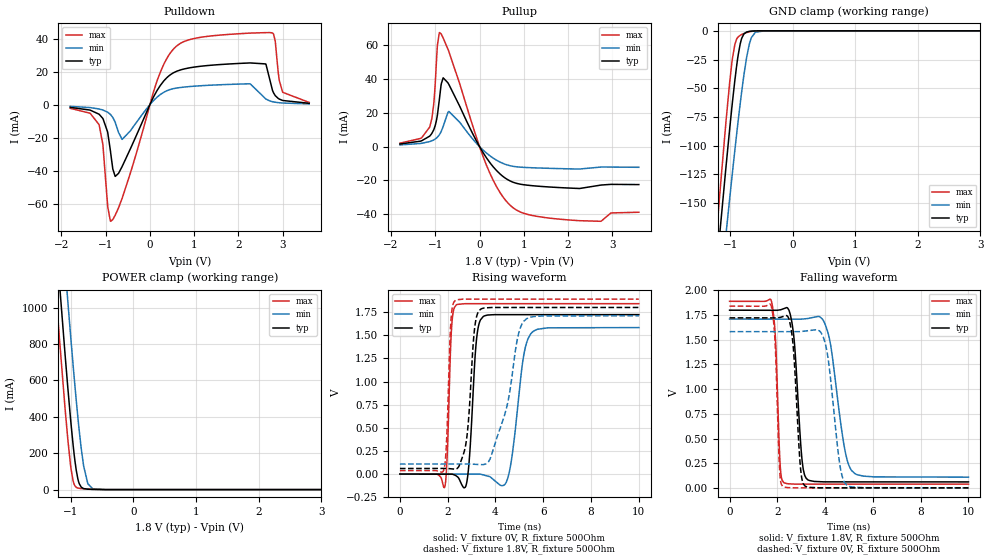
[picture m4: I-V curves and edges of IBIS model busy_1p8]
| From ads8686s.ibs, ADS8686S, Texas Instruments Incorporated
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|   busy_1p8 Model
[Model]   busy_1p8
Model_type   3-state
Polarity   Non-Inverting
Vmeas = 0.9
Vref = 0.9
Cref = 15pF
Rref = 50
|   typ   min   max
C_comp   1.54pF   1.54pF   1.57pF
[Voltage Range]   1.8   1.71   1.89
[Temperature Range]   27   125   -40
[Pullup Reference]   1.8   1.71   1.89
[Pulldown Reference]   0   0   0
[Power Clamp Reference]   1.8   1.71   1.89
[GND Clamp Reference]   0   0   0
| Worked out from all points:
|   slope of the pulldown table from 0 to 0.27 V, typ, clamps not added: 21 ohm
|   slope of the pullup table from 0 to 0.27 V, typ, clamps not added: 25.2 ohm
|   GND clamp passes 1 mA (typ) near -0.73 V on its own axis
|   POWER clamp passes 1 mA (typ) near -0.62 V on its own axis
|   falling waveform, V_fixture 1.8V, R_fixture 500Ohm: 20-80 % time 269ps typ, 526ps min, 163ps max; typ from 1.8 V to 0.06 V
|   rising waveform, V_fixture 0V, R_fixture 500Ohm: 20-80 % time 225ps typ, 418ps min, 136ps max; typ from 0 V to 1.72 V
|   rising waveform, V_fixture 1.8V, R_fixture 500Ohm: 20-80 % time 275ps typ, 761ps min, 144ps max; typ from 0.06 V to 1.8 V
|   falling waveform, V_fixture 0V, R_fixture 500Ohm: 20-80 % time 242ps typ, 420ps min, 155ps max; typ from 1.72 V to 0 V
[Pulldown]
|   Voltage   I(typ)   I(min)   I(max)
-1.8V     -1.668mA   -1.055mA   -2.243mA
-1.152V   -5.772mA   -2.622mA   -12.02mA
-1.066V   -8.317mA   -3.247mA   -23.73mA
-887.4mV  -29.11mA   -6.095mA   -70.65mA
-709.2mV  -41.64mA   -16.83mA   -62.51mA
230.4mV   11.41mA    6.006mA    19.3mA
689.4mV   20.98mA    10.36mA    37.1mA
2.266V    25.24mA    12.61mA    43.3mA
2.617V    24.64mA    3.483mA    43.58mA
2.768V    8.842mA    1.774mA    43.4mA
3.001V    2.503mA    964.9uA    7.472mA
3.6V      800.2uA    430.1uA    1.306mA
[GND Clamp]
|   Voltage   I(typ)   I(min)   I(max)
-1.8V     -573.6mA   -588.4mA   -587.9mA
-1.211V   -204.4mA   -255.9mA   -173.3mA
-1.152V   -168.7mA   -223.4mA   -133.6mA
-1.066V   -118.1mA   -176.9mA   -78.49mA
-1.006V   -84.82mA   -145.6mA   -44.35mA
-968.4mV  -64.72mA   -126.1mA   -26.18mA
-925.2mV  -43.39mA   -104.3mA   -11.96mA
-838.8mV  -11.34mA   -63.25mA   -3.907mA
-779.4mV  -2.722mA   -38.26mA   -2.331mA
-693mV    -444.3uA   -11.52mA   -838.6uA
-595.8mV  -67.67uA   -1.155mA   -139.8uA
3.6V      0A         0A         0A
[Pullup]
|   Voltage   I(typ)   I(min)   I(max)
-1.8V     1.542mA    1.017mA    2.04mA
-1.336V   3.252mA    1.88mA     4.844mA
-1.13V    6.161mA    2.965mA    11.47mA
-1.039V   9.826mA    3.95mA     24.5mA
-952.2mV  18.85mA    5.621mA    60.35mA
-903.6mV  29.12mA    7.211mA    67.66mA
-822.6mV  40.83mA    11.98mA    64.46mA
-693mV    36.85mA    20.85mA    56.33mA
144mV     -6.171mA   -3.541mA   -10.24mA
689.4mV   -20.34mA   -11.32mA   -34.72mA
2.261V    -24.83mA   -13.29mA   -43.94mA
3.6V      -22.51mA   -12.26mA   -38.91mA
[POWER Clamp]
|   Voltage   I(typ)   I(min)   I(max)
-1.8V     4.061A     4.54A      3.768A
-1.233V   1.367A     1.858A     1.061A
-1.179V   1.123A     1.613A     817.9mA
-1.049V   564.5mA    1.04A      280.1mA
-995.4mV  355.2mA    812.6mA    109.9mA
-963mV    243.1mA    681mA      46.78mA
-914.4mV  108.2mA    493.5mA    12.79mA
-865.8mV  32.73mA    323.4mA    7.075mA
-795.6mV  5.598mA    130.2mA    4.664mA
-730.8mV  2.41mA     35.35mA    3.08mA
-649.8mV  1.154mA    4.788mA    1.533mA
3.6V      0A         0A         0A
[Ramp]
R_load = 500
|   typ   min   max
dV/dt_r   1.03354/2.25321e-10   0.949547/4.15937e-10   1.10446/1.36045e-10
dV/dt_f   1.0439/2.69053e-10   0.960924/5.26345e-10   1.11143/1.63233e-10
[Falling Waveform]
V_fixture = 1.8V
V_fixture_min = 1.71V
V_fixture_max = 1.89V
R_fixture = 500Ohm
C_fixture = 0F
|   Time   V(typ)   V(min)   V(max)
0s        1.8V       1.71V      1.89V
1.755ns   1.799V     1.709V     1.888V
2.12ns    1.803V     1.709V     220.4mV
2.258ns   1.815V     1.709V     56.15mV
2.629ns   1.646V     1.709V     39.03mV
3.025ns   302.7mV    1.71V      37.93mV
3.273ns   82.13mV    1.716V     37.92mV
4.095ns   60.71mV    1.591V     37.88mV
5.107ns   60.62mV    175.8mV    37.84mV
10ns      60.17mV    108.5mV    37.61mV
[Rising Waveform]
V_fixture = 0V
V_fixture_min = 0V
V_fixture_max = 0V
R_fixture = 500Ohm
C_fixture = 0F
|   Time   V(typ)   V(min)   V(max)
0s        -48.08nV   -43.12nV   -18.17nV
1.879ns   -678.5uV   -46.34uV   -136.9mV
2.166ns   -782.1uV   -53.41uV   1.598V
2.361ns   -20.42mV   -58.19uV   1.828V
2.808ns   -74.59mV   -69.22uV   1.841V
3.206ns   1.457V     -79.03uV   1.841V
3.49ns    1.703V     -8.848mV   1.841V
4.513ns   1.722V     -45.25mV   1.841V
5.537ns   1.722V     1.533V     1.841V
10ns      1.723V     1.583V     1.841V
[Rising Waveform]
V_fixture = 1.8V
V_fixture_min = 1.71V
V_fixture_max = 1.89V
R_fixture = 500Ohm
C_fixture = 0F
|   Time   V(typ)   V(min)   V(max)
0s        60.17mV    108.5mV    37.61mV
1.838ns   60.95mV    108.8mV    44.75mV
2.135ns   57.32mV    108.8mV    1.658V
2.33ns    54.14mV    108.8mV    1.879V
2.784ns   365.1mV    108.9mV    1.89V
3.112ns   1.542V     106.1mV    1.89V
3.37ns    1.779V     102.7mV    1.89V
4.365ns   1.8V       623.5mV    1.89V
5.189ns   1.8V       1.652V     1.89V
10ns      1.8V       1.71V      1.89V
[Falling Waveform]
|Gnd
V_fixture = 0V
V_fixture_min = 0V
V_fixture_max = 0V
R_fixture = 500Ohm
C_fixture = 0F
|   Time   V(typ)   V(min)   V(max)
0s        1.723V     1.583V     1.841V
1.755ns   1.722V     1.583V     1.835V
2.096ns   1.726V     1.583V     176.4mV
2.217ns   1.734V     1.582V     16.59mV
2.604ns   1.565V     1.582V     1.221mV
2.971ns   196.4mV    1.583V     158uV
3.152ns   19.99mV    1.588V     154uV
3.974ns   536.6uV    1.489V     135.5uV
4.911ns   453.1uV    27.13mV    114.4uV
10ns      -37.44nV   -51.23nV   -54.31nV
